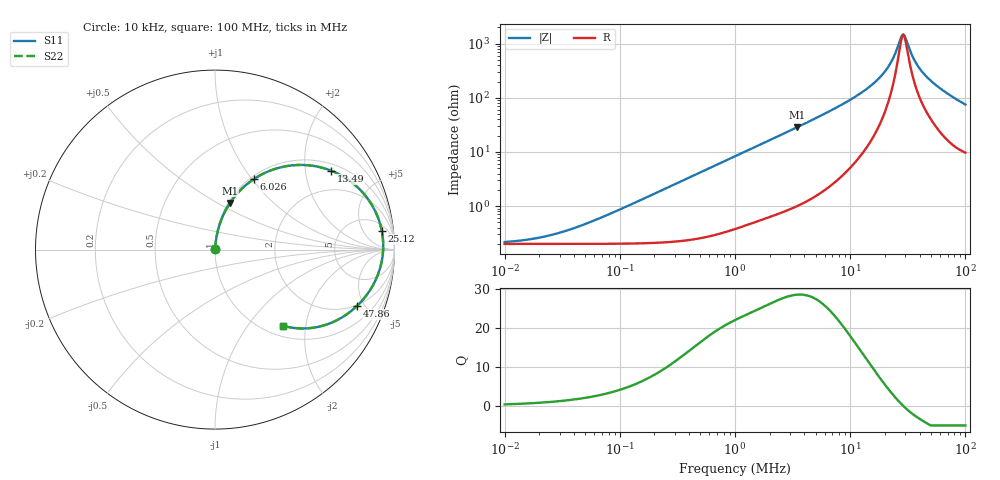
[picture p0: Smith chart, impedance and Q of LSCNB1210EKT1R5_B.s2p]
! LSCNB1210EKT1R5_B  S-PARAMETER MODEL  ( Standard Model )
! Model Generated by TAIYO YUDEN Corporation (http://www.ty-top.com)
! Version 1.0
! TAIYO YUDEN Control No. 191108
! Copyright(c) 2019 TAIYO YUDEN CO.,LTD. All Rights Reserved.
! Product Description (link to TY-COMPAS)
! https://ds.yuden.co.jp/TYCOMPAS/or/detail?pn=LSCNB1210EKT1R5MB&u=M
! Products Name : Inductors
! Characteristics :
!  Inductance : 1.5 [uH] , SRF(min) : - [Hz] , DC Resistance(max) : 240 [mOhm]
!  Rated Current : Saturation  1.2 [A] (dL = 30 [%]), Temp Rise  0.9 [A] (dT = 40 [degC])
!  Case Size : 1.25 x 1.05 / 0.049 x 0.041 [mm/inch] , Thickness : 0.5 / 0.02 [mm/inch]
!  (Conditions: Temperature = 25 [degC] , DC Bias Current = 0 [A])
! External Node Assignments :
!  1  o---GGG---o  2
! GND o---------o GND
! Frequency Range : 10kHz  -  100MHz  [ 402 STEP ]
# MHz S RI R 50
! Freq[MHz].  S11 Real  S11 Imag  S21 Real  S21 Imag  S12 Real  S12 Imag  S22 Real  S22 Imag
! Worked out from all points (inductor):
!   401 points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, 10 kHz to 100 MHz, reference 50 ohm
!   read as one part in series: L = 1.34 uH near 72.44 kHz
!   highest Q = 28.7 at 3.467 MHz (marker M1), where L = 1.32 uH
!   self-resonance near 28.95 MHz
!   S11 on the Smith chart (normalised r, x): 10 kHz: 1.00, +0.00; 6.026 MHz: 1.04, +1.02; 13.49 MHz: 1.22, +2.78; 25.12 MHz: 8, +13; 47.86 MHz: 1.94, -4.43; 100 MHz: 1.19, -1.49
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0.01  0.002 0.000837  0.998 -0.000837  0.998 -0.000837  0.002 0.000837
0.021878  0.002 0.00183  0.998 -0.00183  0.998 -0.00183  0.002 0.00183
0.046774  0.00201 0.00392  0.998 -0.00392  0.998 -0.00392  0.00201 0.00392
0.218776  0.00244 0.0183  0.9976 -0.0183  0.9976 -0.0183  0.00244 0.0183
1  0.0106 0.0821  0.9894 -0.0821  0.9894 -0.0821  0.0106 0.0821
1.905461  0.0297 0.1517  0.9703 -0.1517  0.9703 -0.1517  0.0297 0.1517
3.467369  0.0838 0.2602  0.9162 -0.2602  0.9162 -0.2602  0.0838 0.2602
4.677351  0.1412 0.3308  0.8588 -0.3308  0.8588 -0.3308  0.1412 0.3308
6.025596  0.2164 0.3929  0.7836 -0.3929  0.7836 -0.3929  0.2164 0.3929
9.549926  0.4336 0.4697  0.5664 -0.4697  0.5664 -0.4697  0.4336 0.4697
13.48963  0.6491 0.439  0.3509 -0.439  0.3509 -0.439  0.6491 0.439
17.78279  0.8111 0.3306  0.1889 -0.3306  0.1889 -0.3306  0.8111 0.3306
21.87762  0.8974 0.2037  0.1026 -0.2037  0.1026 -0.2037  0.8974 0.2037
25.11886  0.929 0.1051  0.071 -0.1051  0.071 -0.1051  0.929 0.1051
27.54229  0.9369 0.0367  0.0631 -0.0367  0.0631 -0.0367  0.9369 0.0367
28.84032  0.9369 0.00249  0.0631 -0.00249  0.0631 -0.00249  0.9369 0.00249
29.51209  0.9359 -0.0145  0.0641 0.0145  0.0641 0.0145  0.9359 -0.0145
37.15352  0.8928 -0.174  0.1072 0.174  0.1072 0.174  0.8928 -0.174
41.68694  0.8526 -0.2426  0.1474 0.2426  0.1474 0.2426  0.8526 -0.2426
47.86301  0.7921 -0.313  0.2079 0.313  0.2079 0.313  0.7921 -0.313
69.1831  0.5865 -0.4278  0.4135 0.4278  0.4135 0.4278  0.5865 -0.4278
100  0.3766 -0.4237  0.6234 0.4237  0.6234 0.4237  0.3766 -0.4237
